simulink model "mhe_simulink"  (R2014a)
settings: Solver=ode45  StartTime=0.0  StopTime=100  RelTol=1e-3
libraries: simulink x1

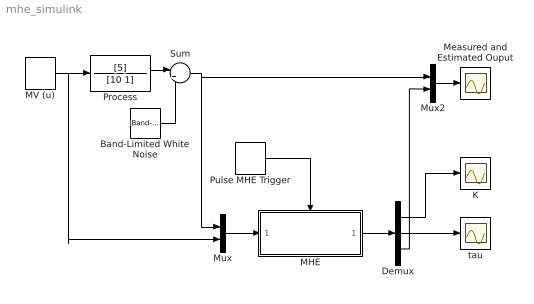
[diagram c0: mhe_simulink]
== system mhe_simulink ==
  Band-Limited White Noise : simulink/Sources/Band-Limited White Noise  Cov=[0.001]  Ts=1.0  seed=[23341]
  Demux : Demux  Outputs=3
  K : Scope
  MHE : Subsystem  TreatAsAtomicUnit=on
  MV (u) : DiscretePulseGenerator  PulseType=Time based  Amplitude=10  Period=50  PulseWidth=30
  Measured and Estimated Ouput : Scope
  Mux : Mux  Inputs=2
  Mux2 : Mux  Inputs=2
  Process : TransferFcn  Numerator=[5]  Denominator=[10 1]
  Pulse MHE Trigger : DiscretePulseGenerator  PulseType=Time based  Period=1  PulseWidth=5
  Sum : Sum  Inputs=|++
  tau : Scope
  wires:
  Process/1 -> Sum/1
  Band-Limited White Noise/1 -> Sum/2
  Sum/1 -> Mux/1, Mux2/1
  Mux/1 -> MHE/1(In1)
  Pulse MHE Trigger/1 -> MHE/Trigger
  MV (u)/1 -> Mux/2, Process/1
  MHE/1(Out1) -> Demux/1
  Demux/1 -> K/1
  Demux/2 -> tau/1
  Mux2/1 -> Measured and Estimated Ouput/1
  Demux/3 -> Mux2/2

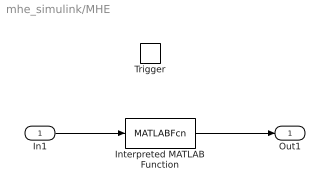
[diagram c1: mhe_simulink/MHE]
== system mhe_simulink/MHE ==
  In1 : Inport
  Trigger : TriggerPort
  Interpreted MATLAB Function : MATLABFcn  MATLABFcn=mhe  OutputDimensions=3
  Out1 : Outport  InitialOutput=[1 10 0]
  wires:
  In1/1 -> Interpreted MATLAB Function/1
  Interpreted MATLAB Function/1 -> Out1/1
